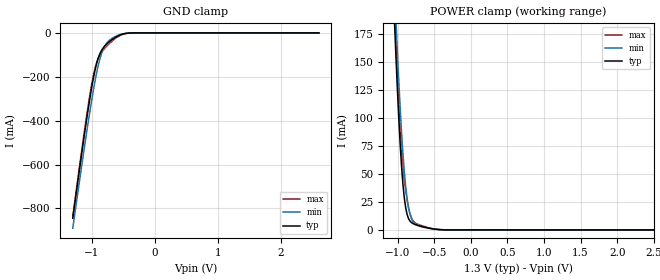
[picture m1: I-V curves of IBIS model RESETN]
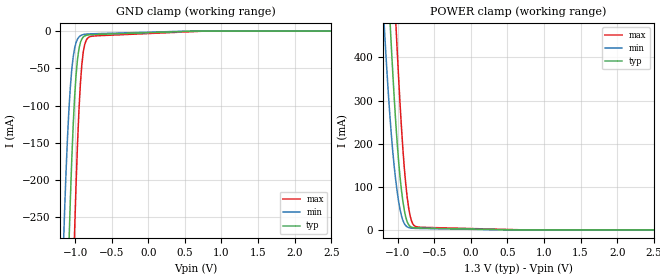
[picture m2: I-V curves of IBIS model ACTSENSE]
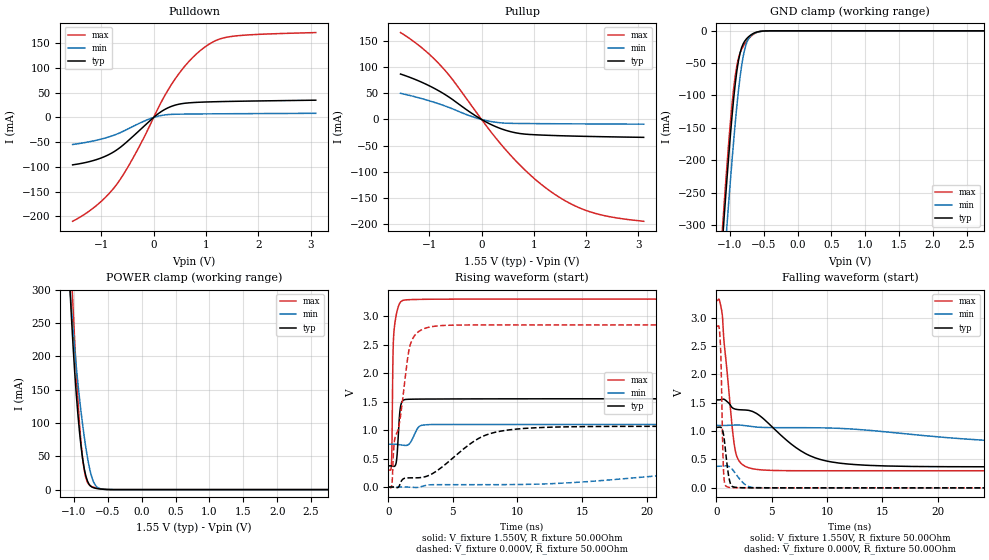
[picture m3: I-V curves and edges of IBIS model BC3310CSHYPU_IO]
| Texas Instruments Incorporated
| Mixed Signal Controller
| Marketing part#   Voltage Range   Package-type   Temperature
| AFE4110AXPFC   1.1V - 3.44V   80-pin LQFP   0 to 85C
| AFE4110B000YS   1.1V - 3.44V   55-pin Bare Die   0 to 85C
[IBIS Ver]   4.0
[File name]   afe4110.ibs
[File Rev]   1.0
[Date]   01/30/2012
[Source]   Model built from TISPICE simulations at:
   Texas Instruments Incorporated.
   Analog-eLab, HPA
   12500 TI Blvd
   Dallas, TX -75243
   For Support e-mail: elab_scm_ibis@list.ti.com
[Notes]   Rev 1.0: 02/03/2012
   - Model based on v1.1 IBIS model for TUSB8040 dated 11/29/2011
   - Model generated from simulations in TISPICED
   - C_comp although listed in numerical order of value are obtained from varying
   PVT conditions. For PVT conditions for each specific value refer the buffer
   description under respective [Model]. IBIS model user is responsible for using
   appropriate C_comp to simulate for Signal Integrity
   Where for TUSB8040
   Nom PVT:  Nominal process, Typ Temperature, Typ Voltage
   Slow PVT: Weak process, Max Temperature, Min Voltage
   Fast PVT: Strong process, Min Temperatire, Max Voltage
[Disclaimer] This product is designed as an aid for customers of Texas Instruments.
   No warranties, either expressed or implied, with respect to this third
   party software (if any) or with respect to its fitness for any
   particular purpose is claimed by Texas Instruments or the author. The
   software (if any) is provided solely on an "as is" basis. The entire
   risk as to its quality and performance is with the customer
[Copyright]   (C)Copyright 2012 Texas Instruments Incorporated.
   All rights reserved.
|   AFE4110A LQFP
[Component]   AFE4110AXPFC
[Manufacturer]  Texas Instruments Incorporated
[Package]   |80-pin LQFP
|   typ   min   max
R_pkg   0.1619   0.1314   0.1841
L_pkg   6.1119nH   5.4033nH   6.8532nH
C_pkg   0.8717pF   0.7514pF   1.1405pF
[PIN]   signal_name   model_name   R_pin   L_pin   C_pin
1   P3P4   CMP09V   0.18405   6.80495nH   0.81165pF
2   P3P5   CMP09V   0.17859   6.5557nH   0.936pF
3   RSTNMI   RESETN   0.1739   6.37029nH   0.9161pF
4   P3P6   BC3310CSHYPU_IO   0.16993   6.20162nH   0.89178pF
5   P3P7   BC3310CSHYPU_IO   0.16665   6.0621nH   0.86995pF
6   VDDIO   POWER   0.16391   5.95909nH   0.79162pF
7   P2P0   BC3325CSHYPU_IO   0.16153   5.80716nH   0.78331pF
8   P2P1   BC3325CSHYPU_IO   0.15992   5.69522nH   0.8313pF
9   P2P2   BC3325CSHYPU_IO   0.1609   6.85318nH   1.14054pF
10   P2P3   BC3325CSHYPU_IO   0.15828   5.64859nH   0.75258pF
11   P4P0   BC3325CSHYPU_IO   0.15761   5.6352nH   0.75136pF
12   P4P1   BC3325CSHYPU_IO   0.15887   6.81175nH   1.13677pF
13   P4P2   BC3325CSHYPU_IO   0.15655   5.62606nH   0.82541pF
14   P4P3   BC3325CSHYPU_IO   0.15688   5.71144nH   0.77508pF
15   VSS   GND   0.15797   5.8369nH   0.78094pF
16   LCD_ECOMP0   LCDSEG_IO   0.15942   5.91356nH   0.8573pF
17   LCD_ECOMP1   LCDSEG_IO   0.1615   6.02835nH   0.87691pF
18   LCD_ECOMP2   LCDSEG_IO   0.16425   6.17172nH   0.89855pF
19   LCD_ECOMP3   LCDSEG_IO   0.16777   6.33298nH   0.91643pF
20   LCD_ESEGP0   LCDSEG_IO   0.17205   6.55761nH   0.79455pF
21   LCD_ESEGP1   LCDSEG_IO   0.1636   6.38684nH   0.79374pF
22   LCD_ESEGP2   LCDSEG_IO   0.15192   6.00586nH   0.91079pF
23   LCD_ESEGP3   LCDSEG_IO   0.14117   5.69327nH   0.88079pF
24   LCD_ESEGP4   LCDSEG_IO   0.13141   5.4033nH   0.82264pF
25   NC   NC   0.00597   3.04786nH   0.64633pF
26   NC   NC   0.00584   2.99862nH   0.57061pF
27   NC   NC   0.0055   2.88531nH   0.56469pF
28   NC   NC   0.00541   2.80573nH   0.61498pF
29   NC   NC   0.00742   3.98553nH   0.92582pF
30   NC   NC   0.00536   2.79276nH   0.53915pF
31   NC   NC   0.00536   2.79307nH   0.5392pF
32   NC   NC   0.00742   3.98612nH   0.92609pF
33   NC   NC   0.00541   2.80659nH   0.61507pF
34   NC   NC   0.0055   2.88609nH   0.56475pF
35   NC   NC   0.00583   2.99598nH   0.56992pF
36   VSS   GND   0.12605   5.21765nH   0.79803pF
37   LCD_ESEGP5   LCDSEG_IO   0.13464   5.46732nH   0.85206pF
38   LCD_ESEGP6   LCDSEG_IO   0.14426   5.75361nH   0.88456pF
39   LCD_ESEGP7   LCDSEG_IO   0.15485   6.06281nH   0.91218pF
40   LCD_ESEGP8   LCDSEG_IO   0.16639   6.43945nH   0.79592pF
41   LCD_ESEGP9   LCDSEG_IO   0.17395   6.5978nH   0.79738pF
42   LCD_ESEGP10   LCDSEG_IO   0.16942   6.36782nH   0.91943pF
43   LCD_ESEGP11   LCDSEG_IO   0.16573   6.20292nH   0.90121pF
44   LCD_EHVCAP   POWER   0.16273   6.05412nH   0.87912pF
45   CP18CAP   NC   0.16042   5.93464nH   0.85913pF
46   CP1P8_C2_IN   NC   0.15875   5.85347nH   0.78233pF
47   CP1P8_C2_OUT   NC   0.15743   5.72309nH   0.7759pF
48   CP1P8_C1_IN   NC   0.15688   5.63318nH   0.82587pF
49   CP1P8_C1_OUT   NC   0.15896   6.8135nH   1.13724pF
50   VPP   NC   0.15748   5.63244nH   0.75124pF
51   P1P0   CMP09V_CMD   0.15792   5.64087nH   0.75183pF
52   P1P1   CMP09V_CMD   0.16032   6.83901nH   1.1395pF
53   P1P2   CMP09V_CMD   0.15913   5.67701nH   0.8299pF
54   P1P3   CMP09V_CMD   0.16053   5.78353nH   0.78165pF
55   P1P4   CMP09V_CMD   0.16271   5.93407nH   0.78941pF
56   P1P5   CMP09V   0.16523   6.03244nH   0.86782pF
57   P1P6   CMP09V   0.16839   6.16946nH   0.88936pF
58   P3P3   CMP09V_CMD   0.17217   6.33401nH   0.91297pF
59   P3P2   CMP09V   0.17669   6.51606nH   0.93253pF
60   ACTIVE   ACTSENSE   0.18195   6.76068nH   0.80905pF
61   VBAT   NC   0.17797   6.67561nH   0.80888pF
62   VSS   GND   0.16698   6.30932nH   0.92591pF
63   VDD   POWER   0.15694   6.01091nH   0.86822pF
64   NC   NC   0.00608   3.11757nH   0.66177pF
65   NC   NC   0.00595   3.04425nH   0.64463pF
66   NC   NC   0.00583   2.99602nH   0.56986pF
67   NC   NC   0.00536   2.86106nH   0.5609pF
68   NC   NC   0.00532   2.79061nH   0.60735pF
69   NC   NC   0.00733   3.97085nH   0.9182pF
70   NC   NC   0.00533   2.78774nH   0.53745pF
71   NC   NC   0.00536   2.79295nH   0.53912pF
72   NC   NC   0.00742   3.98532nH   0.92605pF
73   NC   NC   0.00541   2.80581nH   0.6152pF
74   NC   NC   0.0055   2.88532nH   0.56484pF
75   NC   NC   0.0058   2.99068nH   0.57118pF
76   NC   NC   0.00591   3.03491nH   0.64624pF
77   NC   NC   0.00601   3.10423nH   0.66164pF
78   P3P0   IOSCL15SHY_IO   0.15724   6.00238nH   0.86011pF
79   P3P1   OOSCL15SHY_IO   0.16887   6.33091nH   0.91779pF
80   VSS   GND   0.1802   6.70117nH   0.80766pF
|   AFE4110B000YS Bare Die
[Component]   AFE4110BY000YS
[Manufacturer]  Texas Instruments Incorporated
[Package]   |55-pin bare die
|   typ   min   max
R_pkg   0.001m   0.001m   0.001m
L_pkg   0.001nH   0.001nH   0.001nH
C_pkg   0.001pF   0.001pF   0.001pF
[PIN]   signal_name   model_name   R_pin   L_pin   C_pin
1   P3P0Xin   IOSCL15SHY_IO
2   P3P1Xout   OOSCL15SHY_IO
3   VSS   GND
4   P3P4   CMP09V
5   P3P5   CMP09V
6   RSTNM   RESETN
7   P3P6   BC3310CSHYPU_IO
8   P3P7   BC3310CSHYPU_IO
9   VDDIO   POWER
10   P2P0   BC3325CSHYPU_IO
11   P2P1   BC3325CSHYPU_IO
12   P2P2   BC3325CSHYPU_IO
13   P2P3   BC3325CSHYPU_IO
14   P4P0   BC3325CSHYPU_IO
15   P4P1   BC3325CSHYPU_IO
16   P4P2   BC3325CSHYPU_IO
17   P4P3   BC3325CSHYPU_IO
18   VSS   GND
19   LCD_COM0   LCDSEG_IO
20   LCD_COM1   LCDSEG_IO
21   LCD_COM2   LCDSEG_IO
22   LCD_COM3   LCDSEG_IO
23   LCD_SEG0   LCDSEG_IO
24   LCD_SEG1   LCDSEG_IO
25   LCD_SEG2   LCDSEG_IO
26   LCD_SEG3   LCDSEG_IO
27   LCD_SEG4   LCDSEG_IO
28   VSS   GND
29   LCD_SEG5   LCDSEG_IO
30   LCD_SEG6   LCDSEG_IO
31   LCD_SEG7   LCDSEG_IO
32   LCD_SEG8   LCDSEG_IO
33   LCD_SEG9   LCDSEG_IO
34   LCD_SEG10   LCDSEG_IO
35   LCD_SEG11   LCDSEG_IO
36   CAP   NC
37   CAP   NC
38   C2_IN   NC
39   C2_OUT   NC
40   C1_IN   NC
41   C1_OUT   NC
42   VPP   NC
43   P1P0   CMP09V_CMD
44   P1P1   CMP09V_CMD
45   P1P2   CMP09V_CMD
46   P1P3   CMP09V_CMD
47   P1P4   CMP09V_CMD
48   P1P5   CMP09V
49   P1P6   CMP09V
50   P3P3   CMP09V_CMD
51   P3P2   CMP09V
52   SENSE   ACTSENSE
53   VBAT   NC
54   VSS   GND
55   VDD   POWER
| Models and submodels in the file (9): RESETN (Input), ACTSENSE (Input), BC3310CSHYPU_IO (I/O), BC3325CSHYPU_IO (I/O), CMP09V (I/O), CMP09V_CMD (I/O), IOSCL15SHY_IO (Input), OOSCL15SHY_IO (Input), LCDSEG_IO (I/O)
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|   RESETN Input model
[Model]   RESETN
Model_type   Input
Vinl =  0.39V |0.275V for 1.1V
Vinh =  0.91V |0.825V for 1.1V
|   typ   min   max
|   (weak)   (typ)   (fast)
C_comp   0.7792pF   0.7756pF   0.7828pF
[Model Spec]
Vinl   0.39V   0.275V   0.465V
Vinh   0.91V   0.825V   1.085V
[Voltage Range]   1.300V   1.100V   1.550V
[Temperature Range]   27.0   85.0   0.0
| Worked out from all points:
|   GND clamp passes 1 mA (typ) near -0.42 V on its own axis
|   POWER clamp passes 1 mA (typ) near -0.52 V on its own axis
[GND Clamp]
|   Voltage   I(typ)   I(min)   I(max)
-1.3V     -845.2mA   -890mA     -836.4mA
-1.182V   -599.5mA   -653.6mA   -585.5mA
-1.084V   -402.5mA   -462mA     -385.6mA
-1.026V   -292.7mA   -352.4mA   -276.1mA
-966.8mV  -196.6mA   -250.9mA   -184.9mA
-908mV    -125.2mA   -163.6mA   -124.2mA
-849.2mV  -82.6mA    -98.89mA   -90.41mA
-790.5mV  -58.8mA    -58.92mA   -69.47mA
-712.1mV  -38.29mA   -31.66mA   -46.82mA
-535.7mV  -7.965mA   -6.689mA   -9.902mA
-378.9mV  -410.6uA   -401.1uA   -524.8uA
2.6V      0A         0A         0A
[POWER Clamp]
|   Voltage   I(typ)   I(min)   I(max)
-1.3V     673.1mA    684.4mA    699mA
-1.045V   190.9mA    222.2mA    206.2mA
-1.026V   159.5mA    192.1mA    174.3mA
-1.006V   130mA      163.4mA    144.4mA
-966.8mV  78.74mA    111.5mA    93.68mA
-927.6mV  41.24mA    68.99mA    57.66mA
-908mV    28.45mA    52.06mA    44.8mA
-868.8mV  13.5mA     27.37mA    26.16mA
-810.1mV  6.517mA    9.885mA    10.71mA
-712.1mV  3.812mA    3.572mA    4.78mA
-398.5mV  154.7uA    187.5uA    190.9uA
2.6V      -36.78uA   -23.84uA   -58.74uA
|   ACTSENSE model
[Model]   ACTSENSE
Model_type   Input
Vinl =  0.39V |0.275V for 1.1V
Vinh =  0.91V |0.825V for 1.1V
|   typ   min   max
|   (NOM)   (WEAK)   (FAST)
C_comp   0.5341pF   0.4322pF   0.6511pF
[Model Spec]
Vinl   0.39V   0.275V   0.465V
Vinh   0.91V   0.825V   1.085V
[Voltage Range]   1.300V   1.100V   1.550V
[Temperature Range]   27.0   85.0   0.0
[GND Clamp]
|   Voltage   I(typ)   I(min)   I(max)
-1.3V     -1.206A    -841.9mA   -1.567A
-1.163V   -586mA     -300.1mA   -914mA
-1.143V   -505.6mA   -241.3mA   -824.7mA
-1.084V   -288.3mA   -105.9mA   -567.4mA
-1.045V   -172.3mA   -51.6mA    -408.8mA
-1.006V   -87.89mA   -22.91mA   -267.2mA
-966.8mV  -37.63mA   -10.74mA   -151.4mA
-927.6mV  -15.38mA   -6.265mA   -70.93mA
-908mV    -10.58mA   -5.275mA   -45.22mA
-868.8mV  -6.517mA   -4.321mA   -18.09mA
-770.9mV  -4.788mA   -3.666mA   -6.897mA
2.6V      0A         0A         0A
[POWER Clamp]
|   Voltage   I(typ)   I(min)   I(max)
-1.3V     1.196A     857mA      1.537A
-1.182V   758.4mA    473.7mA    1.071A
-1.104V   485.9mA    262.1mA    769.6mA
-1.084V   422.3mA    218.8mA    696.5mA
-1.026V   250.8mA    115.5mA    485.2mA
-1.006V   202.7mA    89.19mA    418.5mA
-947.2mV  92.31mA    32.99mA    238.2mA
-908mV    45.48mA    14.62mA    143.7mA
-868.8mV  18.84mA    7.185mA    75.92mA
-810.1mV  6.563mA    4.241mA    21.07mA
-712.1mV  4.578mA    3.499mA    6.609mA
2.6V      0A         0A         0A
|   BC3310CSHYPU_IO model
[Model]   BC3310CSHYPU_IO
Model_type   I/O
Vinl = 0.465V  |0.275V for 1.1V
Vinh = 1.085V  |0.825V for 1.1V
Vmeas = 0.755V
Cref = 25pF   |15pF for 1.1V
|   typ   min   max
|   (NOM)   (WEAK)   (FAST)
C_comp   1.9304pF   1.785pF   1.9393pF
[Model Spec]
Vinl   0.465V   0.275V   0.99V
Vinh   1.085V   0.825V   2.31V
[Voltage Range]   1.550V   1.100V   3.300V
[Temperature Range]   27.0   85.0   0.0
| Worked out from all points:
|   slope of the pulldown table from 0 to 0.232 V, typ, clamps not added: 13.5 ohm
|   slope of the pullup table from 0 to 0.232 V, typ, clamps not added: 19.4 ohm
|   GND clamp passes 1 mA (typ) near -0.56 V on its own axis
|   POWER clamp passes 1 mA (typ) near -0.62 V on its own axis
|   falling waveform, V_fixture 1.550V, R_fixture 50.00Ohm: 20-80 % time 4.43ns typ, 13.2ns min, 881ps max; typ from 1.55 V to 0.372 V
|   rising waveform, V_fixture 1.550V, R_fixture 50.00Ohm: 20-80 % time 197ps typ, 456ps min, 136ps max; typ from 0.372 V to 1.55 V
|   rising waveform, V_fixture 0.000V, R_fixture 50.00Ohm: 20-80 % time 3.76ns typ, 13.7ns min, 1.12ns max; typ from 0 V to 1.07 V
|   falling waveform, V_fixture 0.000V, R_fixture 50.00Ohm: 20-80 % time 396ps typ, 954ps min, 184ps max; typ from 1.07 V to 0 V
[Pulldown]
|   Voltage   I(typ)   I(min)   I(max)
-1.55V    -95.73mA   -54.66mA   -209.7mA
-1.106V   -85.55mA   -46.31mA   -178.8mA
-895.7mV  -76.98mA   -40.57mA   -158.5mA
-708.8mV  -65.8mA    -33.83mA   -135.4mA
-334.9mV  -32.36mA   -14.95mA   -70.56mA
202.5mV   15.51mA    4.917mA    42.16mA
389.4mV   24.16mA    6.367mA    74.42mA
576.4mV   28.38mA    6.744mA    101.1mA
950.3mV   31.01mA    7.143mA    139.9mA
1.184V    31.75mA    7.318mA    155.1mA
1.464V    32.39mA    7.496mA    163.2mA
3.1V      34.85mA    8.344mA    171.4mA
[GND Clamp]
|   Voltage   I(typ)   I(min)   I(max)
-1.55V    -1.036A    -1.084A    -1.034A
-1.106V   -321.2mA   -392mA     -301.3mA
-1.083V   -286.7mA   -358.1mA   -266.3mA
-1.036V   -220.2mA   -292mA     -199.1mA
-989.2mV  -158.3mA   -228.6mA   -138.2mA
-942.5mV  -104mA     -169.2mA   -88.16mA
-872.4mV  -46.19mA   -92.36mA   -42.44mA
-825.6mV  -25.88mA   -53.94mA   -28.54mA
-778.9mV  -15.79mA   -28.09mA   -20mA
-662.1mV  -4.562mA   -5.238mA   -6.145mA
-428.4mV  -78.08uA   -144.2uA   -87.52uA
3.1V      0A         0A         0A
[Pullup]
|   Voltage   I(typ)   I(min)   I(max)
-1.55V    86.71mA    49.96mA    165.9mA
-1.106V   69.32mA    38.78mA    133.7mA
-755.5mV  51.05mA    27.77mA    100mA
-545.2mV  37.36mA    19.87mA    74.9mA
-124.6mV  7.656mA    3.579mA    17.09mA
272.6mV   -13.73mA   -5.313mA   -35.41mA
739.9mV   -26.87mA   -7.614mA   -87.67mA
1.207V    -29.97mA   -7.994mA   -129mA
1.651V    -31.4mA    -8.273mA   -158mA
2.072V    -32.39mA   -8.495mA   -176.1mA
2.563V    -33.29mA   -8.719mA   -187.5mA
3.1V      -34.09mA   -8.935mA   -194.3mA
[POWER Clamp]
|   Voltage   I(typ)   I(min)   I(max)
-1.55V    1.479A     1.374A     1.61A
-1.059V   300.8mA    303.2mA    374mA
-1.036V   255.7mA    270.1mA    321.5mA
-1.013V   214mA      239.4mA    270.7mA
-965.8mV  142.7mA    184.4mA    176.7mA
-919.1mV  87.18mA    137.4mA    99.18mA
-872.4mV  46.3mA     97.54mA    46.2mA
-825.6mV  20.84mA    63.54mA    17.87mA
-732.2mV  3.716mA    17.1mA     4.191mA
-662.1mV  1.628mA    4.02mA     2.221mA
-521.9mV  207.3uA    264.7uA    302.3uA
3.1V      0A         0A         -207.8pA
[Ramp]
R_load = 50.00Ohm
|   typ   min   max
dV/dt_r   639.448mV/3.758ns   227.754mV/13.633ns   1.708V/1.116ns
dV/dt_f   706.673mV/4.425ns   208.759mV/13.140ns   1.799V/879.020ps
[Falling Waveform]
V_fixture = 1.550V
V_fixture_min = 1.100V
V_fixture_max = 3.300V
R_fixture = 50.00Ohm
|   Time   V(typ)   V(min)   V(max)
0s        1.55V      1.1V       3.3V
260ps     1.55V      1.1V       3.319V
530ps     1.561V     1.1V       3.068V
1.4ns     1.421V     1.104V     1.143V
1.76ns    1.385V     1.106V     617.6mV
3.7ns     1.302V     1.069V     324.2mV
8.47ns    564.9mV    1.059V     301.5mV
13.92ns   395.1mV    1.012V     301.5mV
36.06ns   371.9mV    765.7mV    301.5mV
125ns     372.2mV    752mV      301.5mV
[Rising Waveform]
V_fixture = 1.550V
V_fixture_min = 1.100V
V_fixture_max = 3.300V
R_fixture = 50.00Ohm
|   Time   V(typ)   V(min)   V(max)
0s        372.2mV    752mV      301.5mV
250ps     370mV      753.3mV    464.7mV
280ps     368.6mV    753.4mV    776.4mV
360ps     364.8mV    753.5mV    2.321V
450ps     363.2mV    753mV      2.772V
650ps     501.5mV    749.1mV    3.065V
950ps     1.421V     740.7mV    3.252V
1.33ns    1.538V     730.8mV    3.286V
3.44ns    1.546V     1.098V     3.298V
125ns     1.55V      1.1V       3.3V
[Rising Waveform]
V_fixture = 0.000V
V_fixture_min = 0.000V
V_fixture_max = 0.000V
R_fixture = 50.00Ohm
|   Time   V(typ)   V(min)   V(max)
0s        71.6uV     110.6uV    24.66uV
260ps     627.8uV    83.9uV     30.8mV
470ps     -818.9uV   298.9uV    807.4mV
870ps     33.53mV    388uV      1.14V
1.7ns     161.8mV    -2.482mV   2.504V
3.76ns    285.1mV    42.27mV    2.829V
7.53ns    911.4mV    42.31mV    2.846V
12.86ns   1.053V     61.84mV    2.846V
37.62ns   1.066V     367.8mV    2.846V
125ns     1.066V     379.7mV    2.846V
[Falling Waveform]
V_fixture = 0.000V
V_fixture_min = 0.000V
V_fixture_max = 0.000V
R_fixture = 50.00Ohm
|   Time   V(typ)   V(min)   V(max)
0s        1.066V     379.7mV    2.846V
240ps     1.069V     380.6mV    2.842V
360ps     1.069V     382.1mV    2.576V
430ps     1.063V     383mV      2.215V
600ps     989.7mV    385.1mV    601.6mV
700ps     881.2mV    386.6mV    161.5mV
1.22ns    113.1mV    369.1mV    7.116mV
2.73ns    2.04mV     42.38mV    851.5uV
4.27ns    1.361mV    2.593mV    216uV
125ns     71.6uV     110.6uV    24.66uV
